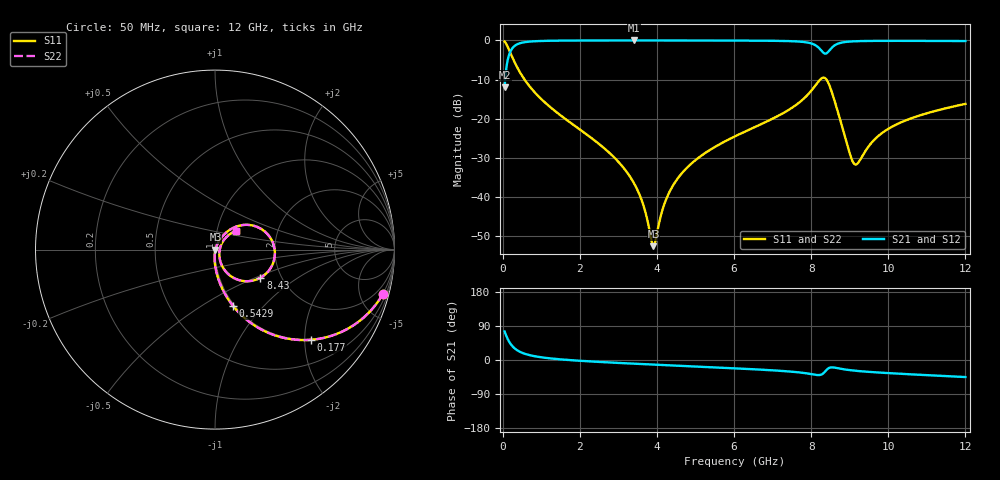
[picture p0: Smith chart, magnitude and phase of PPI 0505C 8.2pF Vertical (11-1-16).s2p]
# GHz S MA R 50
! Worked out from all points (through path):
!   1601 points, 50 MHz to 12 GHz, reference 50 ohm
!   highest |S21| = -0.02 dB at 3.411 GHz (marker M1); lowest = -12.0 dB at 50 MHz (marker M2)
!   group delay of S21, straight-line fit = 13.8 ps
!   lowest |S11| = -52.5 dB at 3.911 GHz (marker M3), VSWR 1.00, Z = 50.2 - j0.0525 ohm
!   |S11| at or under -10 dB: 566.8 MHz to 8.235 GHz (7.668 GHz wide, 174 % of centre); 8.398 GHz to end of sweep
!   |S22| runs from -52.5 to -0.3 dB; largest |S21 - S12| = 0
!   S11 on the Smith chart (normalised r, x): 50 MHz: 0.99, -7.61; 177 MHz: 0.98, -2.15; 542.9 MHz: 0.98, -0.69; 8.43 GHz: 1.57, -0.54; 12 GHz: 1.23, +0.26
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0.05  0.9675 -14.7  0.2517 75.2  0.2517 75.2  0.9675 -14.7
0.1769688  0.7349 -43.1  0.6766 46.7  0.6766 46.7  0.7349 -43.1
0.3263437  0.5056 -60.5  0.8615 29.4  0.8615 29.4  0.5056 -60.5
0.5429375  0.3291 -72.3  0.9432 17.5  0.9432 17.5  0.3291 -72.3
1.088156  0.1624 -83.6  0.9854 6.0  0.9854 6.0  0.1624 -83.6
2.044156  0.07031 -91.0  0.9957 -2.3  0.9957 -2.3  0.07031 -91.0
2.903062  0.03165 -93.6  0.9973 -7.2  0.9973 -7.2  0.03165 -93.6
3.410938  0.01485 -91.4  0.9975 -9.7  0.9975 -9.7  0.01485 -91.4
3.642469  0.008055 -84.6  0.9975 -10.9  0.9975 -10.9  0.008055 -84.6
3.911344  0.002361 -12.8  0.9974 -12.1  0.9974 -12.1  0.002361 -12.8
4.038312  0.004259 42.7  0.9973 -12.7  0.9973 -12.7  0.004259 42.7
4.277312  0.01035 62.1  0.9972 -13.8  0.9972 -13.8  0.01035 62.1
4.643281  0.02006 66.8  0.9968 -15.5  0.9968 -15.5  0.02006 66.8
6.025  0.05956 64.3  0.994 -22.0  0.994 -22.0  0.05956 64.3
7.384313  0.1266 54.9  0.98 -29.9  0.98 -29.9  0.1266 54.9
8.019156  0.2328 36.2  0.9088 -37.5  0.9088 -37.5  0.2328 36.2
8.288031  0.3313 1.3  0.7187 -37.3  0.7187 -37.3  0.3313 1.3
8.429937  0.2978 -31.8  0.704 -23.2  0.704 -23.2  0.2978 -31.8
8.676406  0.1302 -64.4  0.9003 -21.4  0.9003 -21.4  0.1302 -64.4
9.124531  0.02634 -17.1  0.9736 -28.1  0.9736 -28.1  0.02634 -17.1
10.01331  0.07491 47.4  0.9863 -34.7  0.9863 -34.7  0.07491 47.4
12  0.1547 42.4  0.9801 -45.0  0.9801 -45.0  0.1547 42.4
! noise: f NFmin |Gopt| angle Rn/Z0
0.05  0.001441  0.9617  0.3249  0.008496
1.372  0.0044  0.7004  4.733  0.00287
2.701  0.007256  0.6528  8.608  0.003955
4.031  0.01002  0.631  12.48  0.005039
5.36  0.0132  0.6297  16.31  0.006558
6.682  0.01916  0.6753  20.18  0.01105
8.012  0.07317  0.886  24.42  0.1332
9.341  0.04105  0.7784  28.39  0.03569
10.67  0.02941  0.6712  31.81  0.01597
12  0.02923  0.639  35.17  0.01395
